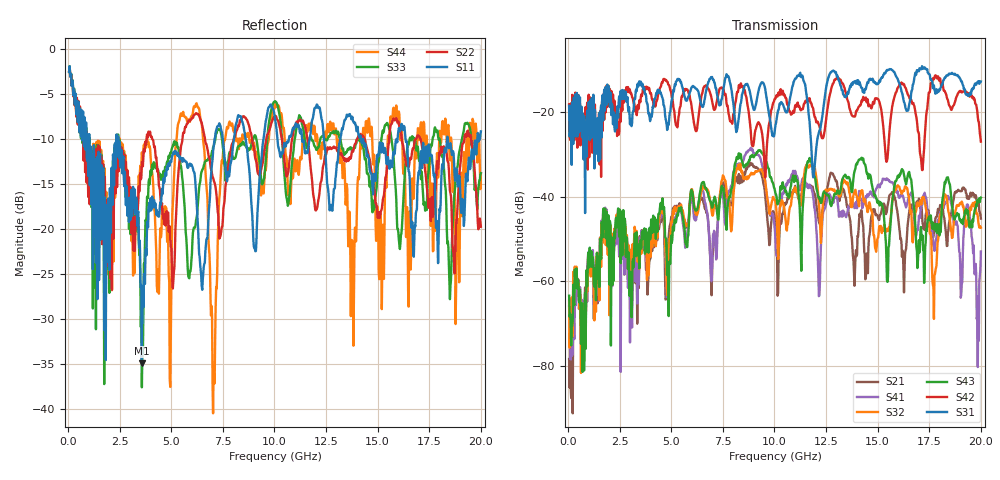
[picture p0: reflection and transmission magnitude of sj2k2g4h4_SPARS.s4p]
! FILE: E:\users\goganessyan\GBX_Backplane\FR408_backplane\1m_OUTBOUND_NEXT\sj2k2g4h4_SPARS.s4p
# MHZ S RI R 50.00
! FREQ  S11  S12  S13  S14
!  S21  S22  S23  S24
!  S31  S32  S33  S34
!  S41  S42  S43  S44
!  REAL  IMAG  REAL  IMAG  REAL  IMAG  REAL  IMAG
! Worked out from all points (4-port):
!   799 points, 50 MHz to 20 GHz, reference 50 ohm
!   strongest paths, dB at 50 MHz, 5.025 GHz, 10.03 GHz, 15.03 GHz, 20 GHz:
!     S31: -18.5, -17.0, -23.9, -13.2, -12.7
!     S42: -18.1, -16.3, -16.7, -16.9, -26.9
!     S43: -63.4, -50.9, -38.6, -40.9, -40.2
!     S32: -64.6, -45.6, -40.7, -49.6, -47.3
!     S41: -65.8, -49.4, -48.1, -37.1, -52.9
!     S21: -78.4, -44.7, -45.3, -45.1, -45.1
!   lowest |S11| = -34.9 dB at 3.575 GHz (marker M1), VSWR 1.04, Z = 48.3 + j0.45 ohm
!   |S11| at or under -10 dB: 2.429 GHz to 7.097 GHz (4.668 GHz wide, 98 % of centre); 14.3 GHz to 15.97 GHz (1.664 GHz wide, 11 % of centre); 16.35 GHz to 18.37 GHz (2.017 GHz wide, 11.6 % of centre)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
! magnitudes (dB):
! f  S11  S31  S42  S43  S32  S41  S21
! 50 MHz  -2.5  -18.5  -18.1  -63.4  -64.6  -65.8  -78.4
! 3.575 GHz  -34.9  -13.9  -16.2  -48.5  -50.3  -48.4  -47.9
! 6.3 GHz  -20.0  -14.9  -21.7  -42.0  -43.4  -42.3  -42.5
! 7.05 GHz  -10.9  -12.3  -19.1  -40.8  -43.0  -48.7  -51.4
! 8.85 GHz  -16.0  -16.2  -24.4  -30.3  -34.7  -28.4  -32.1
! 12.18 GHz  -6.5  -24.3  -23.2  -40.1  -43.1  -63.4  -46.3
! 20 GHz  -9.1  -12.7  -26.9  -40.2  -47.3  -52.9  -45.1
